(* IEC 60870-5-101 balanced mode communication sample (controlling station) *)
PROGRAM P_MAIN_LowSpeed
VAR
	fbClient	: FB_IEC870_5_101M := ( protPara := ( 	linkAddr 	:= 220,(* Link address *)
														eLinkAddrSize := eIEC870_LinkAddr_OneOctet,(* Link address octet size *)
														eLinkMode 	:= eIEC870_LinkMode_Balanced,(* Enable balanced mode *) 
														tClass1Poll := T#100MS,(* Class 1 data poll cycle (high priority) *)
														tClass2Poll := T#100MS ),(* Class 2 data poll cycle (low priority) *) 
										sysPara := ( 	asduAddr 	:= 7,(* Common ASDU address *) 
														nOrg 		:= 0,(* Originator address *)
														bTest		:= TRUE,(* Enable/disable cyclic test command *)
														tTest		:= T#10S,(* Test command cycle time *)
														bClock		:= TRUE,(* Enable/disable cyclic clock synchronisation command *)
														tClock		:= T#20S,(* Clock synchronisation cycle time *)
														bGenin		:= TRUE,(* Enable/disable cyclic general interrogation command *)
														eGeninQoi	:= eIEC870_QOI_INROGEN,(* Qualifier of general interrogation command *)
														tGenin		:= T#40S,(* General interrogation cycle time *)
														bCoro		:= TRUE,(* Enable/disable general counter interrogation command *)														
														eCoroMode 	:= eIEC870_CoroMode_A,(* Counter interrogation mode *)
														bCoroReset	:= FALSE,(* TRUE => Enable reset of counter values (Freeze and reset) *)
														eCoroRqt	:= eIEC870_RQT_REQCOGEN,(* Request qualifier of counter interrogation command *)
														tCoro		:= T#60S,(* Counter interrogation cycle time *)
														bDbgLink 	:= FALSE,(* Enable/disable serial link layer debug messages *)
														bDbgAppl 	:= TRUE,(* Enable/disable application debug messages *)
														eDbgAsdu 	:= eIEC870_FIFO_DBG_OFF,(* Enable/disable ASDU debug messages *)
														asduFmt 	:= ( 	eCOTSize 		:= eIEC870_COT_OneOctet, 
																			eAsduAddrSize 	:= eIEC870_AsduAddr_OneOctet, 
																			eObjAddrSize 	:= eIEC870_ObjAddr_TwoOctets ) 
													) 
									);
										
	stProcData 		: ST_IEC870_5_101MProcData;(* Process data send to or received from IEC 60870-5-101 slave device *)
	fbLog			: FB_IEC870_DebugLogFifo;(* Simple log buffer. We store/log here all our received slave data and other messages *)
	
	bSimulate 	: BOOL := FALSE;(* TRUE => Enable simulation of command data *)
	fbSimulate	: TON := ( IN := FALSE, PT := T#60S );
	bSelect		: BOOL := FALSE;(* TRUE => Select only, FALSE => Execute command *)
END_VAR

(* Execute all master instance fb's *)
fbClient( hSerial := P_SerialComm_HighSpeed.hSerial, stProcData := stProcData, fbLog := fbLog );

(* Simulate command data change *)
fbSimulate( IN := bSimulate );
IF fbSimulate.Q THEN
	fbSimulate( IN := FALSE );
	fbSimulate( IN := bSimulate );

	stProcData.eScs10	:= SEL( stProcData.eScs10 = eIEC870_SCS_OFF, eIEC870_SCS_OFF, eIEC870_SCS_ON );
	stProcData.eQu10 	:= SEL( stProcData.eQu10 = eIEC870_QU_UNSPECIFIED, eIEC870_QU_UNSPECIFIED, eIEC870_QU_SHORTPULSE );
	stProcData.eCtrl10 	:= SEL( bSelect, eIEC870_CMD_EXECUTE, eIEC870_CMD_SELECT );

	stProcData.eDcs20	:= SEL( stProcData.eDcs20 = eIEC870_DCS_OFF, eIEC870_DCS_OFF, eIEC870_DCS_ON );
	stProcData.eQu20 	:= SEL( stProcData.eQu20 = eIEC870_QU_UNSPECIFIED, eIEC870_QU_UNSPECIFIED, eIEC870_QU_SHORTPULSE );
	stProcData.eCtrl20 	:= SEL( bSelect, eIEC870_CMD_EXECUTE, eIEC870_CMD_SELECT );

	stProcData.eRcs30 	:= eIEC870_RCS_INCREMENT;
	stProcData.eQu30 	:= SEL( stProcData.eQu30 = eIEC870_QU_UNSPECIFIED, eIEC870_QU_UNSPECIFIED, eIEC870_QU_SHORTPULSE );
	stProcData.eCtrl30 	:= SEL( bSelect, eIEC870_CMD_EXECUTE, eIEC870_CMD_SELECT );

	stProcData.nBsi40	:= stProcData.nBsi40 + 1;
	stProcData.eCtrl40 	:= eIEC870_CMD_EXECUTE;

	stProcData.nNva50	:= stProcData.nNva50 + 1;
	stProcData.eQl50	:= SEL( stProcData.eQl50 = eIEC870_QL_DEFAULT, eIEC870_QL_DEFAULT, 64 );
	stProcData.eCtrl50 	:= SEL( bSelect, eIEC870_CMD_EXECUTE, eIEC870_CMD_SELECT );

	stProcData.nSva60	:= stProcData.nSva60 + 1;
	stProcData.eQl60	:= SEL( stProcData.eQl60 = eIEC870_QL_DEFAULT, eIEC870_QL_DEFAULT, 64 );
	stProcData.eCtrl60 	:= SEL( bSelect, eIEC870_CMD_EXECUTE, eIEC870_CMD_SELECT );

	stProcData.fSingle70:= stProcData.fSingle70 + 1;
	stProcData.eQl70	:= SEL( stProcData.eQl70 = eIEC870_QL_DEFAULT, eIEC870_QL_DEFAULT, 64 );
	stProcData.eCtrl70 	:= SEL( bSelect, eIEC870_CMD_EXECUTE, eIEC870_CMD_SELECT );
END_IF

END_PROGRAM
